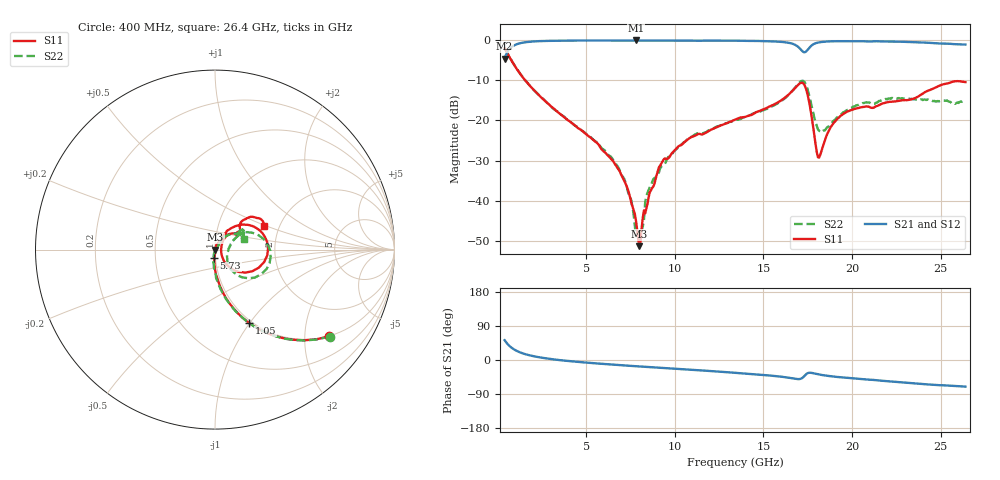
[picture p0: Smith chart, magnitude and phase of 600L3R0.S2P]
!  American Technical Ceramics  Date:  10/27/06
!  One Norden Lane
!  Huntington Station,  NY.  11746-2102
!  Tel:  (631) 622-4700  Fax:  (631) 622-4748
!  Part Number  600L3R0		Mounting Orientation: Vertical
!  Description: Ultra Low ESR Microwave capacitors
!  Application: Coupling, Bypass, Tuning, DC Block
!  Filters, Matching
# GHZ S DB R 50
! Freq  |S11|  S11 Ph  |S21|  S21 Ph  |S12|  S12 Ph  |S22|  S22 Ph
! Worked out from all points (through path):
!   401 points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, 400 MHz to 26.4 GHz, reference 50 ohm
!   highest |S21| = -0.02 dB at 7.81 GHz (marker M1); lowest = -4.5 dB at 400 MHz (marker M2)
!   group delay of S21, straight-line fit = 8.98 ps
!   lowest |S11| = -51.4 dB at 8.005 GHz (marker M3), VSWR 1.01, Z = 50.3 - j0.0302 ohm
!   |S11| at or under -10 dB: 1.566 GHz to end of sweep
!   |S22| runs from -48.9 to -1.9 dB; largest |S21 - S12| = 0.0064
!   S11 on the Smith chart (normalised r, x): 400 MHz: 0.99, -2.63; 1.05 GHz: 0.97, -1.00; 5.73 GHz: 0.98, -0.10; 26.4 GHz: 1.67, +0.47
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0.4  -1.96 -37.3  -4.53 52.3  -4.51 52.2  -1.91 -37.1
1.05  -6.90 -64.9  -1.02 24.8  -1.00 24.8  -6.85 -64.8
2.22  -13.17 -81.2  -0.22 8.3  -0.20 8.2  -13.10 -82.1
4.755  -22.52 -92.8  -0.05 -5.9  -0.04 -6.0  -22.50 -97.0
5.73  -26.20 -96.4  -0.06 -9.5  -0.05 -9.7  -25.97 -101.5
7.16  -35.17 -88.8  -0.03 -14.3  -0.04 -14.6  -34.67 -103.7
7.81  -44.94 -57.8  -0.02 -16.4  -0.04 -16.7  -48.88 -69.3
8.005  -51.37 -6.4  -0.03 -17.1  -0.05 -17.4  -48.59 -22.2
8.135  -46.80 33.7  -0.04 -17.5  -0.06 -17.8  -47.39 22.1
8.46  -40.85 73.3  -0.04 -18.4  -0.06 -18.7  -38.03 27.4
9.11  -31.68 74.5  -0.05 -20.6  -0.07 -20.8  -32.93 46.0
10.8  -24.52 59.0  -0.06 -25.6  -0.07 -25.7  -24.40 56.1
13.4  -19.81 58.1  -0.08 -33.7  -0.10 -33.7  -20.00 49.4
16.52  -13.13 39.1  -0.69 -47.4  -0.72 -47.2  -13.15 25.6
17.17  -10.58 1.2  -2.55 -48.2  -2.58 -48.1  -10.10 -7.2
17.43  -12.41 -30.4  -2.70 -36.8  -2.73 -36.7  -11.33 -35.0
17.755  -19.91 -52.2  -1.16 -34.3  -1.19 -34.2  -17.01 -51.4
18.145  -29.28 5.5  -0.50 -38.3  -0.52 -38.2  -22.58 -25.0
18.795  -21.69 50.0  -0.24 -42.8  -0.26 -42.6  -20.78 17.8
19.445  -18.60 47.3  -0.19 -46.0  -0.22 -45.9  -18.27 27.8
22.11  -15.34 36.3  -0.30 -56.3  -0.32 -56.0  -14.48 36.3
26.4  -10.41 25.3  -1.05 -70.3  -1.06 -70.0  -15.25 20.0
